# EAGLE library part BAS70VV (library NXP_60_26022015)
General-purpose Schottky diodes General-purpose Schottky diodes in small Surface-Mounted Device (SMD) plastic packages. AAL Eindhoven MK
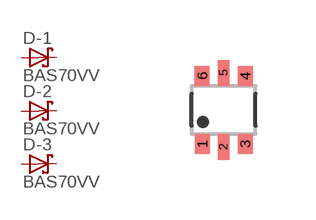
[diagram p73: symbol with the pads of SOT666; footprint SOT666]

Designator prefix D; gates -1=DIODE_SCHOTTKY -2=DIODE_SCHOTTKY -3=DIODE_SCHOTTKY

## BAS70VV  [SOT666]
1  -1:A  pas
2  -2:A  pas
3  -3:A  pas
4  -3:K  pas
5  -2:K  pas
6  -1:K  pas

## Footprint SOT666 (pad centres in mm)
SOT 666 Reflow soldering foorprint Source: Philips - BAS70_1PS7XSB70_SER_8.pdf
smd 0.375 x 0.5: 1 -0.537,-0.85; 3 0.538,-0.85; 4 0.538,0.85; 6 -0.538,0.85
smd 0.3 x 0.65: 2 0,-0.925; 5 0,0.925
